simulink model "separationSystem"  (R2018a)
settings: Solver=ode15s  StartTime=0.0  StopTime=180000  RelTol=1e-5
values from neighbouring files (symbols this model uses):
  d_time = 3600*[2,4,18]    [runSimulation.m]    (also in runSimulation_BulkSep.m = 1e6*[1,1,1])
  e_in_val = 0.15    [init_param.m]    (also in init_param_new.m)
  F_in_val = [0.456,0.59]'    [init_param.m]    (also in init_param_new.m)
  ns_tot = ns_o + ns_w + 3    (= 543)    [init_param.m]    (also in runSimulation.m = ns_w + ns_o + 3; RTO.m = 1010; SS.m = 1010)
  rto_sol_time = 6500000    [runSimulation.m]
  t_filter = 2000    [runSimulation.m]
  Y1_case2 = [x_solution(453); x_solution(451); x_solution(452)]    [runSimulation.m]
  Y1_case2_step = 0*(Y1_case2 - Y1.sp)    [runSimulation.m]
  Y1_case3 = [x_solution(453); x_solution(451); x_solution(452)]    [runSimulation.m]
  Y1_case3_step = 0*(Y1_case3 - Y1_case2)    [runSimulation.m]
undefined symbols (not defined in the file or in its folder): c1, cfu, CFU_model_sim, gs1, GS1_model_sim, hc, HC_model_sim, stepTime, U1_step, Y1
libraries: simulink x4

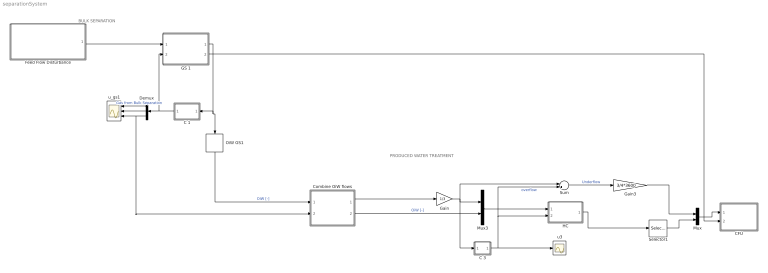
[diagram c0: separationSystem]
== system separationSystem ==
  note: PRODUCED WATER TREATMENT
  note: BULK SEPARATION
  C 1 : Subsystem
  C 3 : Subsystem
  CFU : Subsystem
  Combine OiW flows : Subsystem
  Demux : Demux  Outputs=3
  Feed Flow Disturbance : Subsystem
  GS 1 : Subsystem
  Gain : Gain  Gain=1/3
  Gain3 : Gain  Gain=3/4*3600
  HC : Subsystem
  Mux : Mux  Inputs=2
  Mux3 : Mux  Inputs=2
  OiW GS1 : Selector  InputPortWidth=5  IndexOptions=Index vector (dialog)  Indices=5  OutputSizes=1
  Selector1 : Selector  InputPortWidth=2  IndexOptions=Index vector (dialog)  Indices=[2]  OutputSizes=1
  Sum : Sum  Inputs=|+-
  u3 : Scope
  u_gs1 : Scope  NumInputPorts=3
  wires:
  GS 1/1(Y 1) -> C 1/1(Y 1), OiW GS1/1
  Demux/2 -> u_gs1/2
  C 1/1(U 1) -> GS 1/2(Input), Demux/1
  Demux/1 -> u_gs1/1  "Gas from Bulk Separation"
  C 3/1(U) -> u3/1, Sum/2, HC/2(Input)  "overflow"
  HC/1("Y ") -> Selector1/1
  Mux3/1 -> HC/1(Disturbance)
  Mux/1 -> CFU/1(Disturbance)
  Gain3/1 -> Mux/1
  Sum/1 -> Gain3/1  "Underflow"
  Gain/1 -> Mux3/1, Sum/1, C 3/1(Y)
  OiW GS1/1 -> Combine OiW flows/1("ppm 1 ")  "OiW [-]"
  Demux/3 -> Combine OiW flows/2(flow 1), u_gs1/3
  Feed Flow Disturbance/1(Well Fluids) -> GS 1/1(Disturbance)
  Selector1/1 -> Mux/2
  Combine OiW flows/1(Flow HC feed) -> Gain/1
  Combine OiW flows/2(OiW HC feed) -> Mux3/2  "OiW [-]"
  GS 1/2(Pin) -> CFU/2(Pin)

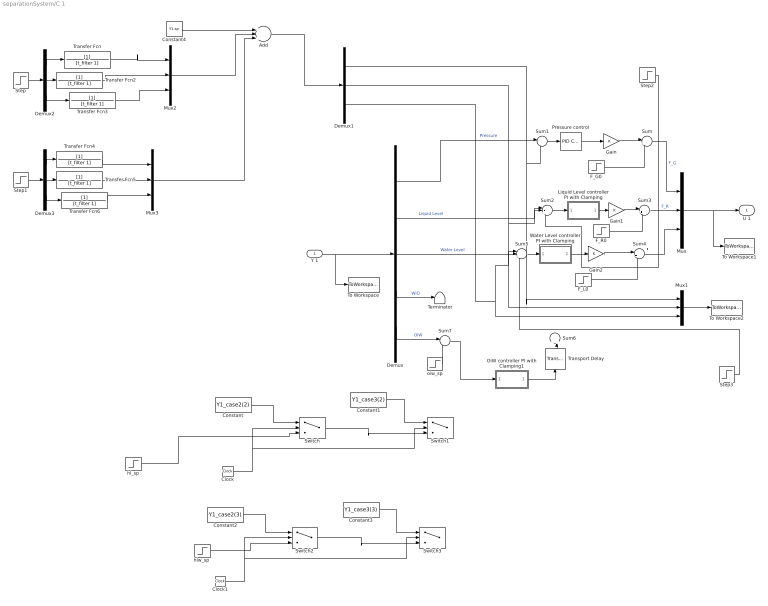
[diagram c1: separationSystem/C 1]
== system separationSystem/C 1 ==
  Y 1 : Inport
  Add : Sum  Inputs=+++
  Clock : Clock
  Clock1 : Clock
  Constant : Constant  Commented=on  Value=Y1_case2(2)
  Constant1 : Constant  Commented=on  Value=Y1_case3(2)
  Constant2 : Constant  Commented=on  Value=Y1_case2(3)
  Constant3 : Constant  Commented=on  Value=Y1_case3(3)
  Constant4 : Constant  Value=Y1.sp
  Demux : Demux  Outputs=5
  Demux1 : Demux  Outputs=3
  Demux2 : Demux  Outputs=3
  Demux3 : Demux  Outputs=3
  F_G0 : Step  Time=stepTime  Before=gs1.U(1)  After=gs1.U(1)*U1_step(1)  SampleTime=0
  F_L0 : Step  Time=stepTime  Before=gs1.U(3)  After=gs1.U(3)*U1_step(3)  SampleTime=0
  F_R0 : Step  Time=stepTime  Before=gs1.U(2)  After=gs1.U(2)*U1_step(2)  SampleTime=0
  Gain : Gain
  Gain1 : Gain
  Gain2 : Gain
  Liquid Level controller PI with Clamping : Subsystem
  Mux{,1..3} (4 alike) : Mux  Inputs=3
  OiW controller PI with Clamping1 : Subsystem  Commented=on
  Pressure control : simulink/Continuous/PID Controller  Controller=PI  TimeDomain=Continuous-time  SampleTime=-1  IntegratorMethod=Forward Euler  FilterMethod=Forward Euler  Form=Parallel  UseFilter=on  ControllerParametersSource=internal  P=-0.1935  I=-0.1935/20  D=0  N=100  InitialConditionSource=internal  InitialConditionForIntegrator=0  InitialConditionForFilter=0  ExternalReset=none  LimitOutput=on  UpperSaturationLimit=inf  LowerSaturationLimit=-gs1.U(1)  LinearizeAsGain=on  AntiWindupMode=none  Kb=1  TrackingMode=off  Kt=1  PParamMin=[]  PParamMax=[]  IParamMin=[]  IParamMax=[]  DParamMin=[]  DParamMax=[]  NParamMin=[]  NParamMax=[]  KbParamMin=[]  KbParamMax=[]  KtParamMin=[]  KtParamMax=[]  POutMin=[]  POutMax=[]  IOutMin=[]  IOutMax=[]  DOutMin=[]  DOutMax=[]  NOutMin=[]  NOutMax=[]  KbOutMin=[]  KbOutMax=[]  KtOutMin=[]  KtOutMax=[]  IntegratorOutMin=[]  IntegratorOutMax=[]  FilterOutMin=[]  FilterOutMax=[]  SumOutMin=[]  SumOutMax=[]  SumI1OutMin=[]  SumI1OutMax=[]  SumI2OutMin=[]  SumI2OutMax=[]  SumI3OutMin=[]  SumI3OutMax=[]  SumDOutMin=[]  SumDOutMax=[]  SaturationOutMin=[]  SaturationOutMax=[]  IntegratorContinuousStateAttributes=''  IntegratorStateMustResolveToSignalObject=off  IntegratorRTWStateStorageClass=Auto  FilterContinuousStateAttributes=''  FilterStateMustResolveToSignalObject=off  FilterRTWStateStorageClass=Auto  DifferentiatorICPrevScaledInput=0  DifferentiatorOutMin=[]  DifferentiatorOutMax=[]  InitialConditionSetting=State (most efficient)  FilterDiffOutCoefMin=[]  FilterDiffOutCoefMax=[]  SumDenOutMin=[]  SumDenOutMax=[]  SumNumOutMin=[]  SumNumOutMax=[]  ReciprocalOutMin=[]  ReciprocalOutMax=[]  DivideOutMin=[]  DivideOutMax=[]  TunerSelectOption=Transfer Function Based (PID Tuner App)
  Step : Step  Time=d_time(2)  After=Y1_case2_step  SampleTime=0
  Step1 : Step  Time=d_time(3)  After=Y1_case3_step  SampleTime=0
  Step2 : Step  Time=126000  After=0.1  SampleTime=0
  Step3 : Step  Time=126000+20000  After=-0.05  SampleTime=0
  Sum : Sum  Inputs=|++
  Sum1 : Sum  Inputs=|-+
  Sum2 : Sum  Inputs=|-++
  Sum3 : Sum  Inputs=|++
  Sum4 : Sum  Inputs=|++
  Sum5 : Sum  Inputs=|-++
  Sum6 : Sum  Commented=on  Inputs=++|
  Sum7 : Sum  Commented=on  Inputs=|-+
  Switch : Switch  Commented=on  Criteria=u2 > Threshold  Threshold=d_time(2)+rto_sol_time
  Switch1 : Switch  Commented=on  Criteria=u2 > Threshold  Threshold=d_time(3)+rto_sol_time
  Switch2 : Switch  Commented=on  Criteria=u2 > Threshold  Threshold=d_time(2)+rto_sol_time
  Switch3 : Switch  Commented=on  Criteria=u2 > Threshold  Threshold=d_time(3)+rto_sol_time
  Terminator : Terminator
  To Workspace : ToWorkspace  VariableName=gs1_Y  SaveFormat=Structure With Time  SampleTime=-1
  To Workspace1 : ToWorkspace  VariableName=gs1_U  SaveFormat=Structure With Time  SampleTime=-1
  To Workspace2 : ToWorkspace  VariableName=gs1_Ysp  SaveFormat=Structure With Time  SampleTime=-1
  Transfer Fcn{,2..6} (6 alike) : TransferFcn  Denominator=[t_filter 1]
  Transport Delay : TransportDelay  Commented=on  DelayTime=0.1
  Water Level controller PI with Clamping : Subsystem
  hl_sp : Step  Commented=on  Time=stepTime  Before=Y1.sp(2)  After=Y1.sp(2)*Y1.step(2)  SampleTime=0
  "hlw_sp " : Step  Commented=on  Time=stepTime  Before=Y1.sp(3)  After=Y1.sp(3)*Y1.step(3)  SampleTime=0
  oiw_sp : Step  Commented=on  Time=stepTime  Before=Y1.sp(4)  After=Y1.sp(4)*Y1.step(4)  SampleTime=0.1
  U 1 : Outport
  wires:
  Sum2/1 -> Liquid Level controller PI with Clamping/1(e)
  Demux1/2 -> Mux1/2, Sum2/2
  Liquid Level controller PI with Clamping/1(delta_u) -> Gain1/1
  Sum5/1 -> Water Level controller PI with Clamping/1(e)
  F_L0/1 -> Sum4/2
  Y 1/1 -> To Workspace/1, Demux/1
  Sum1/1 -> Pressure control/1
  Demux/1 -> Sum1/1  "Pressure"
  Demux1/1 -> Sum1/2, Mux1/1
  Pressure control/1 -> Gain/1
  Mux/1 -> To Workspace1/1, U 1/1
  Demux/2 -> Sum2/1  "Liquid Level"
  Demux/3 -> Sum5/1  "Water Level"
  Water Level controller PI with Clamping/1(delta_u) -> Gain2/1
  Demux/4 -> Terminator/1  "WiO"
  Demux/5 -> Sum7/1  "OiW"
  Sum4/1 -> Mux/3  "F_L"
  Sum3/1 -> Mux/2  "F_R"
  F_R0/1 -> Sum3/2
  F_G0/1 -> Sum/2
  Sum/1 -> Mux/1  "F_G"
  OiW controller PI with Clamping1/1(delta_u) -> Transport Delay/1
  Sum7/1 -> OiW controller PI with Clamping1/1(e)
  oiw_sp/1 -> Sum7/2
  Demux1/3 -> Mux1/3, Sum5/2
  Transport Delay/1 -> Sum6/2
  Mux1/1 -> To Workspace2/1
  Gain/1 -> Sum/1
  Gain1/1 -> Sum3/1
  Gain2/1 -> Sum4/1
  Clock/1 -> Switch/2, Switch1/2
  hl_sp/1 -> Switch/3
  Switch/1 -> Switch1/3
  Constant/1 -> Switch/1
  Constant1/1 -> Switch1/1
  Constant2/1 -> Switch2/1
  Switch2/1 -> Switch3/3
  Constant3/1 -> Switch3/1
  "hlw_sp "/1 -> Switch2/3
  Clock1/1 -> Switch2/2, Switch3/2
  Constant4/1 -> Add/1
  Step/1 -> Demux2/1
  Step1/1 -> Demux3/1
  Mux2/1 -> Add/2
  Mux3/1 -> Add/3
  Add/1 -> Demux1/1
  Demux2/1 -> Transfer Fcn/1
  Demux2/2 -> Transfer Fcn2/1
  Demux2/3 -> Transfer Fcn3/1
  Demux3/1 -> Transfer Fcn4/1
  Demux3/2 -> Transfer Fcn5/1
  Demux3/3 -> Transfer Fcn6/1
  Transfer Fcn/1 -> Mux2/1
  Transfer Fcn2/1 -> Mux2/2
  Transfer Fcn3/1 -> Mux2/3
  Transfer Fcn4/1 -> Mux3/1
  Transfer Fcn5/1 -> Mux3/2
  Transfer Fcn6/1 -> Mux3/3
  Step2/1 -> Sum2/3
  Step3/1 -> Sum5/3

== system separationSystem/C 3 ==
  Y : Inport
  Constant4 : Constant  Value=hc.sp
  Multiply : Product
  To Workspace2 : ToWorkspace  VariableName=hc_U  SaveFormat=Structure With Time  SampleTime=-1
  U : Outport
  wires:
  Y/1 -> Multiply/2  "inflow"
  Multiply/1 -> To Workspace2/1, U/1  "Oil outlet flow (Control input)"
  Constant4/1 -> Multiply/1

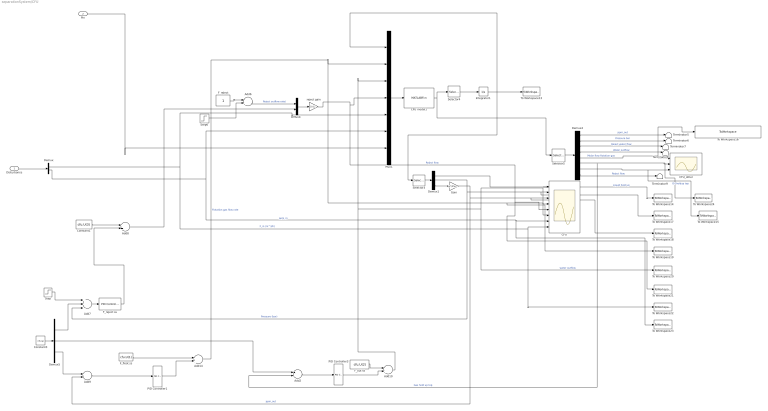
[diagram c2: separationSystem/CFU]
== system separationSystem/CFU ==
  Disturbance : Inport
  Pin : Inport  Port=2
  Add{6,8,10,14} (4 alike) : Sum
  Add2 : Sum  Inputs=+-
  Add7 : Sum  Inputs=++-
  Add9 : Sum  Inputs=+-
  CFU : Scope  NumInputPorts=8
  CFU model1 : MATLABFcn  MATLABFcn=CFU_model_sim(u(1:35),u(36:38),u(39:40),u(41))
  CFU_other : Scope  NumInputPorts=3
  Constant1 : Constant  Value=cfu.U(3)
  Constant3 : Constant  Value=cfu.sp
  Demux : Demux  Outputs=2
  Demux1 : Demux  Outputs=3
  Demux4 : Demux  Outputs=8
  Demux5 : Demux  Outputs=3
  F_float ss : Constant  Value=cfu.U(1)
  F_out ss : Constant  Value=cfu.U(2)
  F_reject : Constant
  F_reject ss : simulink/Continuous/PID Controller  Controller=PI  TimeDomain=Continuous-time  SampleTime=-1  IntegratorMethod=Forward Euler  FilterMethod=Forward Euler  Form=Ideal  UseFilter=on  ControllerParametersSource=internal  P=-36.93/4  I=1/100/4  D=0  N=100  InitialConditionSource=internal  InitialConditionForIntegrator=0  InitialConditionForFilter=0  ExternalReset=none  LimitOutput=off  UpperSaturationLimit=inf  LowerSaturationLimit=0  LinearizeAsGain=on  AntiWindupMode=clamping  Kb=1  TrackingMode=off  Kt=1  PParamMin=[]  PParamMax=[]  IParamMin=[]  IParamMax=[]  DParamMin=[]  DParamMax=[]  NParamMin=[]  NParamMax=[]  KbParamMin=[]  KbParamMax=[]  KtParamMin=[]  KtParamMax=[]  POutMin=[]  POutMax=[]  IOutMin=[]  IOutMax=[]  DOutMin=[]  DOutMax=[]  NOutMin=[]  NOutMax=[]  KbOutMin=[]  KbOutMax=[]  KtOutMin=[]  KtOutMax=[]  IntegratorOutMin=[]  IntegratorOutMax=[]  FilterOutMin=[]  FilterOutMax=[]  SumOutMin=[]  SumOutMax=[]  SumI1OutMin=[]  SumI1OutMax=[]  SumI2OutMin=[]  SumI2OutMax=[]  SumI3OutMin=[]  SumI3OutMax=[]  SumDOutMin=[]  SumDOutMax=[]  SaturationOutMin=[]  SaturationOutMax=[]  IntegratorContinuousStateAttributes=''  IntegratorStateMustResolveToSignalObject=off  IntegratorRTWStateStorageClass=Auto  FilterContinuousStateAttributes=''  FilterStateMustResolveToSignalObject=off  FilterRTWStateStorageClass=Auto  DifferentiatorICPrevScaledInput=0  DifferentiatorOutMin=[]  DifferentiatorOutMax=[]  InitialConditionSetting=State (most efficient)  FilterDiffOutCoefMin=[]  FilterDiffOutCoefMax=[]  SumDenOutMin=[]  SumDenOutMax=[]  SumNumOutMin=[]  SumNumOutMax=[]  ReciprocalOutMin=[]  ReciprocalOutMax=[]  DivideOutMin=[]  DivideOutMax=[]  TunerSelectOption=Transfer Function Based (PID Tuner App)
  Gain : Gain  Gain=pi*(25e-6)^3/6 * 1e10*1e6
  Integrator1 : Integrator  InitialCondition=cfu.x0
  Mux1 : Mux  Inputs=7
  Mux4 : Mux  Inputs=2
  PID Controller1 : simulink/Continuous/PID Controller  Controller=PI  TimeDomain=Continuous-time  SampleTime=-1  IntegratorMethod=Forward Euler  FilterMethod=Forward Euler  Form=Ideal  UseFilter=on  ControllerParametersSource=internal  P=-1.3308/4/5  I=1/100/4/5  D=0  N=100  InitialConditionSource=internal  InitialConditionForIntegrator=0  InitialConditionForFilter=0  ExternalReset=none  LimitOutput=off  UpperSaturationLimit=inf  LowerSaturationLimit=-inf  LinearizeAsGain=on  AntiWindupMode=none  Kb=1  TrackingMode=off  Kt=1  PParamMin=[]  PParamMax=[]  IParamMin=[]  IParamMax=[]  DParamMin=[]  DParamMax=[]  NParamMin=[]  NParamMax=[]  KbParamMin=[]  KbParamMax=[]  KtParamMin=[]  KtParamMax=[]  POutMin=[]  POutMax=[]  IOutMin=[]  IOutMax=[]  DOutMin=[]  DOutMax=[]  NOutMin=[]  NOutMax=[]  KbOutMin=[]  KbOutMax=[]  KtOutMin=[]  KtOutMax=[]  IntegratorOutMin=[]  IntegratorOutMax=[]  FilterOutMin=[]  FilterOutMax=[]  SumOutMin=[]  SumOutMax=[]  SumI1OutMin=[]  SumI1OutMax=[]  SumI2OutMin=[]  SumI2OutMax=[]  SumI3OutMin=[]  SumI3OutMax=[]  SumDOutMin=[]  SumDOutMax=[]  SaturationOutMin=[]  SaturationOutMax=[]  IntegratorContinuousStateAttributes=''  IntegratorStateMustResolveToSignalObject=off  IntegratorRTWStateStorageClass=Auto  FilterContinuousStateAttributes=''  FilterStateMustResolveToSignalObject=off  FilterRTWStateStorageClass=Auto  DifferentiatorICPrevScaledInput=0  DifferentiatorOutMin=[]  DifferentiatorOutMax=[]  InitialConditionSetting=State (most efficient)  FilterDiffOutCoefMin=[]  FilterDiffOutCoefMax=[]  SumDenOutMin=[]  SumDenOutMax=[]  SumNumOutMin=[]  SumNumOutMax=[]  ReciprocalOutMin=[]  ReciprocalOutMax=[]  DivideOutMin=[]  DivideOutMax=[]  TunerSelectOption=Transfer Function Based (PID Tuner App)
  PID Controller3 : simulink/Continuous/PID Controller  Controller=PI  TimeDomain=Continuous-time  SampleTime=-1  IntegratorMethod=Forward Euler  FilterMethod=Forward Euler  Form=Ideal  UseFilter=on  ControllerParametersSource=internal  P=-15.3846  I=1/100  D=0  N=100  InitialConditionSource=internal  InitialConditionForIntegrator=0  InitialConditionForFilter=0  ExternalReset=none  LimitOutput=off  UpperSaturationLimit=inf  LowerSaturationLimit=-inf  LinearizeAsGain=on  AntiWindupMode=none  Kb=1  TrackingMode=off  Kt=1  PParamMin=[]  PParamMax=[]  IParamMin=[]  IParamMax=[]  DParamMin=[]  DParamMax=[]  NParamMin=[]  NParamMax=[]  KbParamMin=[]  KbParamMax=[]  KtParamMin=[]  KtParamMax=[]  POutMin=[]  POutMax=[]  IOutMin=[]  IOutMax=[]  DOutMin=[]  DOutMax=[]  NOutMin=[]  NOutMax=[]  KbOutMin=[]  KbOutMax=[]  KtOutMin=[]  KtOutMax=[]  IntegratorOutMin=[]  IntegratorOutMax=[]  FilterOutMin=[]  FilterOutMax=[]  SumOutMin=[]  SumOutMax=[]  SumI1OutMin=[]  SumI1OutMax=[]  SumI2OutMin=[]  SumI2OutMax=[]  SumI3OutMin=[]  SumI3OutMax=[]  SumDOutMin=[]  SumDOutMax=[]  SaturationOutMin=[]  SaturationOutMax=[]  IntegratorContinuousStateAttributes=''  IntegratorStateMustResolveToSignalObject=off  IntegratorRTWStateStorageClass=Auto  FilterContinuousStateAttributes=''  FilterStateMustResolveToSignalObject=off  FilterRTWStateStorageClass=Auto  DifferentiatorICPrevScaledInput=0  DifferentiatorOutMin=[]  DifferentiatorOutMax=[]  InitialConditionSetting=State (most efficient)  FilterDiffOutCoefMin=[]  FilterDiffOutCoefMax=[]  SumDenOutMin=[]  SumDenOutMax=[]  SumNumOutMin=[]  SumNumOutMax=[]  ReciprocalOutMin=[]  ReciprocalOutMax=[]  DivideOutMin=[]  DivideOutMax=[]  TunerSelectOption=Transfer Function Based (PID Tuner App)
  Selector3 : Selector  InputPortWidth=35  IndexOptions=Index vector (dialog)  Indices=[31 32 33]  OutputSizes=1
  Selector4 : Selector  InputPortWidth=43  IndexOptions=Index vector (dialog)  Indices=[1:35]  OutputSizes=1
  Selector5 : Selector  InputPortWidth=43  IndexOptions=Index vector (dialog)  Indices=[36:43]  OutputSizes=1
  Step : Step  Time=169200+100000  After=-0.05  SampleTime=0
  Step6 : Step  After=0  SampleTime=0
  Terminator{5..9} (5 alike) : Terminator
  To Workspace13 : ToWorkspace  VariableName=x_simulink1  SampleTime=-1
  To Workspace14 : ToWorkspace  VariableName=liq_hold_up1  SampleTime=-1
  To Workspace15 : ToWorkspace  VariableName=oil_hold_up1  SampleTime=-1
  To Workspace16 : ToWorkspace  VariableName=mass_flow_flotation1  SampleTime=-1
  To Workspace17 : ToWorkspace  VariableName=Pressure1  SampleTime=-1
  To Workspace18 : ToWorkspace  VariableName=ppm_out1  SampleTime=-1
  To Workspace19 : ToWorkspace  VariableName=F_flotation1  SampleTime=-1
  To Workspace20 : ToWorkspace  VariableName=F_out1  SampleTime=-1
  To Workspace21 : ToWorkspace  VariableName=F_reject1  SampleTime=-1
  To Workspace22 : ToWorkspace  VariableName=F_in1  SampleTime=-1
  To Workspace23 : ToWorkspace  VariableName=ppm_in1  SampleTime=-1
  To Workspace24 : ToWorkspace  VariableName=gas_hold_up1  SampleTime=-1
  reject gain : Gain  Gain=[0 1]  Multiplication=Matrix(K*u)
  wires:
  Disturbance/1 -> Demux/1
  Add14/1 -> Mux1/2, CFU/6, To Workspace19/1  "Flotation gas flow rate"
  CFU model1/1 -> Selector4/1, Selector5/1
  Demux4/1 -> Terminator5/1  "ppm_out"
  Demux/1 -> Mux1/5, CFU/8, To Workspace22/1  "F_in (m^3/h)"
  Demux4/3 -> Terminator7/1  "Reject water flow"
  Demux1/3 -> Gain/1
  Demux4/4 -> Terminator8/1  "Water outflow"
  Add6/1 -> Mux4/1  "Reject outflow rate)"
  PID Controller1/1 -> Add14/2
  Demux1/1 -> To Workspace14/1, CFU/1  "Liquid hold up"
  F_out ss/1 -> Add10/1
  F_reject/1 -> Add6/1
  Demux4/5 -> To Workspace16/1, CFU_other/1  "Molar flow flotation gas"
  Demux4/7 -> To Workspace15/1, CFU_other/3  "Oil holdup top"
  Demux4/2 -> Terminator6/1  "Pressure bar"
  Selector5/1 -> Demux4/1
  Mux4/1 -> reject gain/1
  Demux1/2 -> Add7/3, CFU/2, To Workspace17/1  "Pressure (bar)"
  reject gain/1 -> CFU/5, To Workspace21/1, Mux1/4  "Reject flow"
  Add8/1 -> Mux4/2
  Step6/1 -> Add6/2
  Gain/1 -> CFU/3, To Workspace18/1, Add9/2  "ppm_out"
  Mux1/1 -> CFU model1/1
  Demux4/8 -> Terminator9/1  "Reject flow"
  Selector3/1 -> Demux1/1
  Integrator1/1 -> To Workspace13/1, Selector3/1, Mux1/1
  F_float ss/1 -> Add14/1
  Selector4/1 -> Integrator1/1
  F_reject ss/1 -> Add8/2
  Demux/2 -> CFU/7, To Workspace23/1, Mux1/6  "ppm_in"
  Constant1/1 -> Add8/1
  Demux4/6 -> Add2/2, To Workspace24/1, CFU_other/2  "Gas hold up top"
  Add9/1 -> PID Controller1/1
  Demux5/1 -> Add7/2
  Demux5/3 -> Add9/1
  Demux5/2 -> Add2/1
  Add7/1 -> F_reject ss/1
  Add10/1 -> Mux1/3, CFU/4, To Workspace20/1  "water outflow"
  Constant3/1 -> Demux5/1
  Add2/1 -> PID Controller3/1
  PID Controller3/1 -> Add10/2
  Pin/1 -> Mux1/7
  Step/1 -> Add7/1

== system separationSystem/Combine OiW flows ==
  "ppm 1 " : Inport
  flow 1 : Inport  Port=2
  Divide : Product  Inputs=*/
  Gain : Gain  Gain=1e-6
  Mux : Mux  Inputs=2
  Product1 : Product
  To Workspace : ToWorkspace  VariableName=D_hc  SaveFormat=Structure With Time  SampleTime=-1
  Flow HC feed : Outport
  OiW HC feed : Outport  Port=2
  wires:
  Product1/1 -> Divide/1  "v1"
  flow 1/1 -> Flow HC feed/1, Mux/1, Divide/2, Product1/2  "v tot"
  "ppm 1 "/1 -> Product1/1
  Divide/1 -> Gain/1
  Mux/1 -> To Workspace/1
  Gain/1 -> Mux/2, OiW HC feed/1

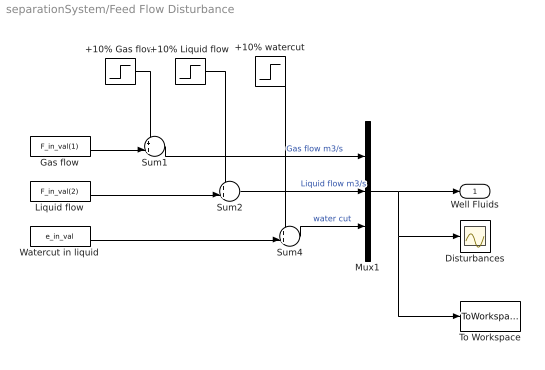
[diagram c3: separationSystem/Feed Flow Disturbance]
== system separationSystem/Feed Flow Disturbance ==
  +10% Gas flow : Step  Time=d_time(1)  After=0.1*F_in_val(1)  SampleTime=0
  +10% Liquid flow : Step  Time=d_time(2)  After=0.1*F_in_val(2)  SampleTime=0
  +10% watercut : Step  Time=d_time(3)  After=0.1*e_in_val  SampleTime=0
  Disturbances : Scope
  Gas flow : Constant  Value=F_in_val(1)
  Liquid flow : Constant  Value=F_in_val(2)
  Mux1 : Mux  Inputs=3
  Sum1 : Sum  Inputs=++|
  Sum2 : Sum  Inputs=++|
  Sum4 : Sum  Inputs=++|
  To Workspace : ToWorkspace  VariableName=simD  SaveFormat=Structure With Time  SampleTime=-1
  Watercut in liquid : Constant  Value=e_in_val
  Well Fluids : Outport
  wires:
  Mux1/1 -> To Workspace/1, Disturbances/1, Well Fluids/1
  Sum2/1 -> Mux1/2  "Liquid flow m3/s"
  Sum4/1 -> Mux1/3  "water cut"
  Liquid flow/1 -> Sum2/2
  Watercut in liquid/1 -> Sum4/2
  +10% Liquid flow/1 -> Sum2/1
  +10% watercut/1 -> Sum4/1
  Sum1/1 -> Mux1/1  "Gas flow m3/s"
  Gas flow/1 -> Sum1/2
  +10% Gas flow/1 -> Sum1/1

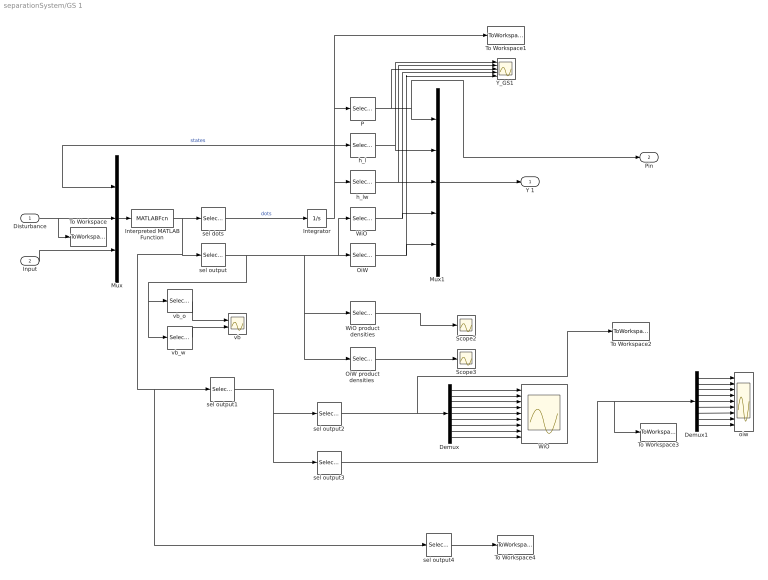
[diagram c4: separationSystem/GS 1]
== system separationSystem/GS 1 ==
  Disturbance : Inport
  Input : Inport  Port=2
  Demux : Demux  Commented=on  Outputs=9
  Demux1 : Demux  Commented=on  Outputs=9
  Integrator : Integrator  InitialCondition=gs1.x0
  Interpreted MATLAB Function : MATLABFcn  MATLABFcn=GS1_model_sim(u(1:ns_tot),u(ns_tot+1:ns_tot+3),u(ns_tot+4:ns_tot+6))
  Mux : Mux  Inputs=3
  Mux1 : Mux  Inputs=5
  OiW : Selector  InputPortWidth=24  IndexOptions=Index vector (dialog)  Indices=[2]  OutputSizes=1
  "OiW product densities " : Selector  InputPortWidth=24  IndexOptions=Index vector (dialog)  Indices=[13:22]  OutputSizes=1
  P : Selector  InputPortWidth=ns_tot  IndexOptions=Index vector (dialog)  Indices=ns_tot  OutputSizes=1
  Scope2 : Scope
  Scope3 : Scope
  To Workspace : ToWorkspace  VariableName=gs1_D  SaveFormat=Structure With Time  SampleTime=-1
  To Workspace1 : ToWorkspace  VariableName=xSol_gs1  SaveFormat=Structure With Time  SampleTime=-1
  To Workspace2 : ToWorkspace  VariableName=wio  SampleTime=-1
  To Workspace3 : ToWorkspace  VariableName=oiw  SampleTime=-1
  To Workspace4 : ToWorkspace  VariableName=rho_all  SampleTime=-1
  WiO : Scope  NumInputPorts=9
  "WiO " : Selector  InputPortWidth=24  IndexOptions=Index vector (dialog)  Indices=[1]  OutputSizes=1
  WiO product densities : Selector  InputPortWidth=24  IndexOptions=Index vector (dialog)  Indices=[3:12]  OutputSizes=1
  "Y_GS1 " : Scope  NumInputPorts=5
  h_l : Selector  InputPortWidth=ns_tot  IndexOptions=Index vector (dialog)  Indices=[ns_tot-2]  OutputSizes=1
  h_lw : Selector  InputPortWidth=ns_tot  IndexOptions=Index vector (dialog)  Indices=[ns_tot-1]  OutputSizes=1
  oiw : Scope  NumInputPorts=9
  sel dots : Selector  InputPortWidth=ns_tot+24+18+180+66+300  IndexOptions=Index vector (dialog)  Indices=[1:ns_tot]  OutputSizes=1
  sel output : Selector  InputPortWidth=ns_tot+24+18+180+66+300  IndexOptions=Index vector (dialog)  Indices=[ns_tot+1:ns_tot+24]  OutputSizes=1
  sel output1 : Selector  InputPortWidth=ns_tot+24+18+180+66+300  IndexOptions=Index vector (dialog)  Indices=[ns_tot+24+1:ns_tot+24+18+6]  OutputSizes=1
  sel output2 : Selector  InputPortWidth=24  IndexOptions=Index vector (dialog)  Indices=[1:12]  OutputSizes=1
  sel output3 : Selector  InputPortWidth=24  IndexOptions=Index vector (dialog)  Indices=[13:24]  OutputSizes=1
  sel output4 : Selector  InputPortWidth=ns_tot+24+18+180+66+300  IndexOptions=Index vector (dialog)  Indices=[ns_tot+24+18+6+1:ns_tot+24+18+180+66+300]  OutputSizes=1
  vb : Scope  NumInputPorts=2
  vb_o : Selector  InputPortWidth=24  IndexOptions=Index vector (dialog)  Indices=[23]  OutputSizes=1
  "vb_w " : Selector  InputPortWidth=24  IndexOptions=Index vector (dialog)  Indices=[24]  OutputSizes=1
  Y 1 : Outport
  Pin : Outport  Port=2
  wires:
  Mux/1 -> Interpreted MATLAB Function/1
  Integrator/1 -> To Workspace1/1, P/1, Mux/1, h_l/1, h_lw/1  "states"
  Interpreted MATLAB Function/1 -> sel output4/1, sel output1/1, sel output/1, sel dots/1
  sel output/1 -> vb_o/1, "vb_w "/1, "OiW product densities "/1, WiO product densities/1, "WiO "/1, OiW/1
  "vb_w "/1 -> vb/2
  vb_o/1 -> vb/1
  Input/1 -> Mux/3
  Disturbance/1 -> To Workspace/1, Mux/2
  Mux1/1 -> Y 1/1
  OiW/1 -> Mux1/5, "Y_GS1 "/5
  WiO product densities/1 -> Scope2/1
  P/1 -> "Y_GS1 "/3, Pin/1, Mux1/1
  h_lw/1 -> "Y_GS1 "/2, Mux1/3
  "WiO "/1 -> Mux1/4, "Y_GS1 "/4
  "OiW product densities "/1 -> Scope3/1
  sel dots/1 -> Integrator/1  "dots"
  h_l/1 -> "Y_GS1 "/1, Mux1/2
  sel output1/1 -> sel output3/1, sel output2/1
  sel output2/1 -> To Workspace2/1, Demux/1
  Demux/1 -> WiO/1
  Demux/2 -> WiO/2
  Demux/3 -> WiO/3
  Demux/4 -> WiO/4
  Demux/5 -> WiO/5
  Demux/6 -> WiO/6
  Demux/7 -> WiO/7
  Demux/8 -> WiO/8
  Demux/9 -> WiO/9
  Demux1/7 -> oiw/7
  Demux1/1 -> oiw/1
  Demux1/4 -> oiw/4
  Demux1/6 -> oiw/6
  Demux1/9 -> oiw/9
  Demux1/3 -> oiw/3
  sel output3/1 -> To Workspace3/1, Demux1/1
  Demux1/8 -> oiw/8
  Demux1/5 -> oiw/5
  Demux1/2 -> oiw/2
  sel output4/1 -> To Workspace4/1

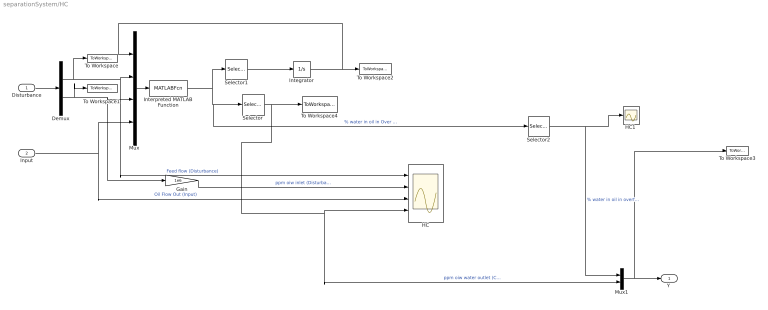
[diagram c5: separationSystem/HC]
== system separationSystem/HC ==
  Disturbance : Inport
  Input : Inport  Port=2
  Demux : Demux  Outputs=2
  Gain : Gain  Gain=1e6
  HC : Scope  NumInputPorts=4
  "HC1 " : Scope
  Integrator : Integrator  InitialCondition=hc.x0
  Interpreted MATLAB Function : MATLABFcn  MATLABFcn=HC_model_sim(u(1:432),u(433),u(434),u(435))
  Mux : Mux
  Mux1 : Mux  Inputs=2
  Selector : Selector  InputPortWidth=436  IndexOptions=Index vector (dialog)  Indices=[435]  OutputSizes=1
  Selector1 : Selector  InputPortWidth=436  IndexOptions=Index vector (dialog)  Indices=[1:432]  OutputSizes=1
  Selector2 : Selector  InputPortWidth=436  IndexOptions=Index vector (dialog)  Indices=[436]  OutputSizes=1
  To Workspace : ToWorkspace  VariableName=F_in_sim  SampleTime=-1
  To Workspace1 : ToWorkspace  VariableName=e_in_sim  SampleTime=-1
  To Workspace2 : ToWorkspace  VariableName=xSol_hc  SaveFormat=Structure With Time  SampleTime=-1
  To Workspace3 : ToWorkspace  VariableName=hc_Y  SaveFormat=Structure With Time  SampleTime=-1
  To Workspace4 : ToWorkspace  VariableName=e_out_sim  SampleTime=-1
  "Y " : Outport
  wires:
  Integrator/1 -> Mux/1, To Workspace2/1
  Selector/1 -> Mux1/2, HC/4, To Workspace4/1  "ppm oiw water outlet (CV)"
  Interpreted MATLAB Function/1 -> Selector1/1, Selector2/1, Selector/1  "% water in oil in Over flow"
  Mux/1 -> Interpreted MATLAB Function/1
  Gain/1 -> HC/2  "ppm oiw inlet (Disturbance)"
  Disturbance/1 -> Demux/1
  Input/1 -> Mux/4, HC/3  "Oil Flow Out (Input)"
  Selector1/1 -> Integrator/1
  Demux/1 -> To Workspace/1, HC/1, Mux/2  "Feed flow (Disturbance)"
  Demux/2 -> To Workspace1/1, Gain/1, Mux/3
  Selector2/1 -> "HC1 "/1, Mux1/1  "% water in oil in overflow"
  Mux1/1 -> To Workspace3/1, "Y "/1

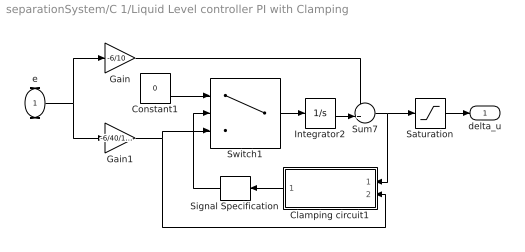
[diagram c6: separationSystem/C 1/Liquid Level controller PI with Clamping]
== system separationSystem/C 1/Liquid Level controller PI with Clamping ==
  e : Inport
  Clamping circuit1 : Subsystem
  Constant1 : Constant  Value=0
  Gain : Gain  Gain=-6/10
  Gain1 : Gain  Gain=-6/40/100
  Integrator2 : Integrator
  Saturation : Saturate  UpperLimit=inf  LowerLimit=-gs1.U(2)
  Signal Specification : SignalSpecification  Dimensions=1
  Sum7 : Sum  Inputs=++|
  Switch1 : Switch  Criteria=u2 > Threshold
  delta_u : Outport
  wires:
  Sum7/1 -> Clamping circuit1/1(preSat), Saturation/1
  Integrator2/1 -> Sum7/2
  Saturation/1 -> delta_u/1
  Switch1/1 -> Integrator2/1
  Constant1/1 -> Switch1/1
  e/1 -> Gain1/1, Gain/1
  Gain1/1 -> Clamping circuit1/2(preIntegrator), Switch1/3
  Gain/1 -> Sum7/1
  Clamping circuit1/1(Clamp) -> Signal Specification/1
  Signal Specification/1 -> Switch1/2

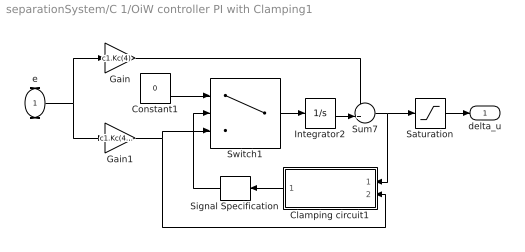
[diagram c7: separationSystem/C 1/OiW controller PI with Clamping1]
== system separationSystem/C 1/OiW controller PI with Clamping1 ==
  e : Inport
  Clamping circuit1 : Subsystem
  Constant1 : Constant  Value=0
  Gain : Gain  Gain=c1.Kc(4)
  Gain1 : Gain  Gain=c1.Kc(4)/c1.taui(4)
  Integrator2 : Integrator
  Saturation : Saturate  UpperLimit=4-Y1.sp(3)  LowerLimit=-Y1.sp(3)
  Signal Specification : SignalSpecification  Dimensions=1
  Sum7 : Sum  Inputs=++|
  Switch1 : Switch  Criteria=u2 > Threshold
  delta_u : Outport
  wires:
  Sum7/1 -> Clamping circuit1/1(preSat), Saturation/1
  Integrator2/1 -> Sum7/2
  Saturation/1 -> delta_u/1
  Switch1/1 -> Integrator2/1
  Constant1/1 -> Switch1/1
  e/1 -> Gain1/1, Gain/1
  Gain1/1 -> Clamping circuit1/2(preIntegrator), Switch1/3
  Gain/1 -> Sum7/1
  Clamping circuit1/1(Clamp) -> Signal Specification/1
  Signal Specification/1 -> Switch1/2

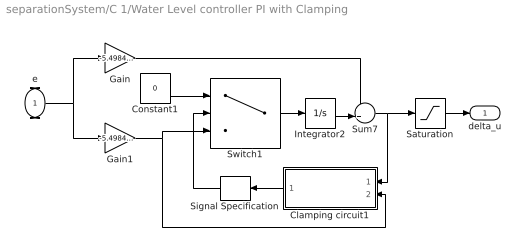
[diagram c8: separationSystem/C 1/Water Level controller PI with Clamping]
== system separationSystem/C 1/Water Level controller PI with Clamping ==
  e : Inport
  Clamping circuit1 : Subsystem
  Constant1 : Constant  Value=0
  Gain : Gain  Gain=-5.4984/200
  Gain1 : Gain  Gain=-5.4984/40/40000
  Integrator2 : Integrator
  Saturation : Saturate  UpperLimit=inf  LowerLimit=-gs1.U(3)
  Signal Specification : SignalSpecification  Dimensions=1
  Sum7 : Sum  Inputs=++|
  Switch1 : Switch  Criteria=u2 > Threshold
  delta_u : Outport
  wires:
  Sum7/1 -> Clamping circuit1/1(preSat), Saturation/1
  Integrator2/1 -> Sum7/2
  Saturation/1 -> delta_u/1
  Switch1/1 -> Integrator2/1
  Constant1/1 -> Switch1/1
  e/1 -> Gain1/1, Gain/1
  Gain1/1 -> Clamping circuit1/2(preIntegrator), Switch1/3
  Gain/1 -> Sum7/1
  Clamping circuit1/1(Clamp) -> Signal Specification/1
  Signal Specification/1 -> Switch1/2

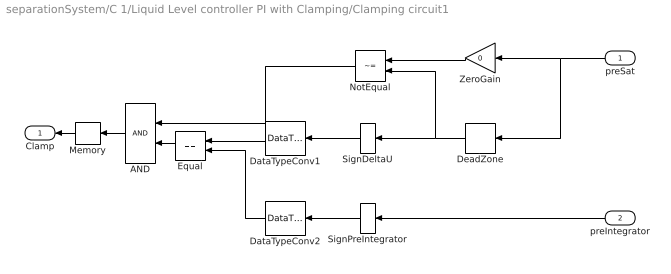
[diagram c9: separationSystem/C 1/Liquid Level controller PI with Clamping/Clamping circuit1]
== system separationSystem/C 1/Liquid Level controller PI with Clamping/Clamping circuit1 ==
  preSat : Inport  DisableCoverage=on
  preIntegrator : Inport  DisableCoverage=on  Port=2
  AND : Logic  DisableCoverage=on
  DataTypeConv1 : DataTypeConversion  DisableCoverage=on  OutDataTypeStr=int8
  DataTypeConv2 : DataTypeConversion  DisableCoverage=on  OutDataTypeStr=int8
  DeadZone : DeadZone  DisableCoverage=on  LowerValue=-gs1.U(2)  UpperValue=inf
  Equal : RelationalOperator  DisableCoverage=on  Operator===
  Memory : Memory  DisableCoverage=on
  NotEqual : RelationalOperator  DisableCoverage=on  Operator=~=
  SignDeltaU : Signum  DisableCoverage=on
  SignPreIntegrator : Signum  DisableCoverage=on
  ZeroGain : Gain  DisableCoverage=on  Gain=0
  Clamp : Outport  DisableCoverage=on
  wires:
  preSat/1 -> ZeroGain/1, DeadZone/1
  preIntegrator/1 -> SignPreIntegrator/1
  ZeroGain/1 -> NotEqual/1
  DeadZone/1 -> NotEqual/2, SignDeltaU/1
  SignDeltaU/1 -> DataTypeConv1/1
  DataTypeConv1/1 -> Equal/1
  SignPreIntegrator/1 -> DataTypeConv2/1
  DataTypeConv2/1 -> Equal/2
  NotEqual/1 -> AND/1
  Equal/1 -> AND/2
  AND/1 -> Memory/1
  Memory/1 -> Clamp/1

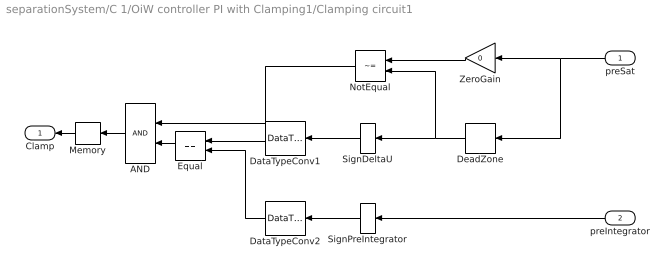
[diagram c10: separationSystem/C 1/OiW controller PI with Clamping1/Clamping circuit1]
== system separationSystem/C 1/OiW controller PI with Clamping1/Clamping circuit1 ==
  preSat : Inport  DisableCoverage=on
  preIntegrator : Inport  DisableCoverage=on  Port=2
  AND : Logic  DisableCoverage=on
  DataTypeConv1 : DataTypeConversion  DisableCoverage=on  OutDataTypeStr=int8
  DataTypeConv2 : DataTypeConversion  DisableCoverage=on  OutDataTypeStr=int8
  DeadZone : DeadZone  DisableCoverage=on  LowerValue=-Y1.sp(3)  UpperValue=4-Y1.sp(3)
  Equal : RelationalOperator  DisableCoverage=on  Operator===
  Memory : Memory  DisableCoverage=on
  NotEqual : RelationalOperator  DisableCoverage=on  Operator=~=
  SignDeltaU : Signum  DisableCoverage=on
  SignPreIntegrator : Signum  DisableCoverage=on
  ZeroGain : Gain  DisableCoverage=on  Gain=0
  Clamp : Outport  DisableCoverage=on
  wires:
  preSat/1 -> ZeroGain/1, DeadZone/1
  preIntegrator/1 -> SignPreIntegrator/1
  ZeroGain/1 -> NotEqual/1
  DeadZone/1 -> NotEqual/2, SignDeltaU/1
  SignDeltaU/1 -> DataTypeConv1/1
  DataTypeConv1/1 -> Equal/1
  SignPreIntegrator/1 -> DataTypeConv2/1
  DataTypeConv2/1 -> Equal/2
  NotEqual/1 -> AND/1
  Equal/1 -> AND/2
  AND/1 -> Memory/1
  Memory/1 -> Clamp/1

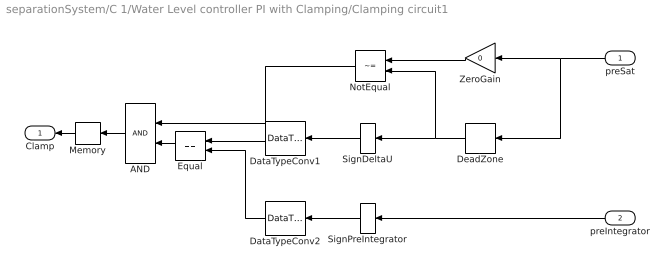
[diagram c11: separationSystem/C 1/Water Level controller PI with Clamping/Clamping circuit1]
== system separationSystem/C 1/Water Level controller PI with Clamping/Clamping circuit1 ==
  preSat : Inport  DisableCoverage=on
  preIntegrator : Inport  DisableCoverage=on  Port=2
  AND : Logic  DisableCoverage=on
  DataTypeConv1 : DataTypeConversion  DisableCoverage=on  OutDataTypeStr=int8
  DataTypeConv2 : DataTypeConversion  DisableCoverage=on  OutDataTypeStr=int8
  DeadZone : DeadZone  DisableCoverage=on  LowerValue=-gs1.U(3)  UpperValue=inf
  Equal : RelationalOperator  DisableCoverage=on  Operator===
  Memory : Memory  DisableCoverage=on
  NotEqual : RelationalOperator  DisableCoverage=on  Operator=~=
  SignDeltaU : Signum  DisableCoverage=on
  SignPreIntegrator : Signum  DisableCoverage=on
  ZeroGain : Gain  DisableCoverage=on  Gain=0
  Clamp : Outport  DisableCoverage=on
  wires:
  preSat/1 -> ZeroGain/1, DeadZone/1
  preIntegrator/1 -> SignPreIntegrator/1
  ZeroGain/1 -> NotEqual/1
  DeadZone/1 -> NotEqual/2, SignDeltaU/1
  SignDeltaU/1 -> DataTypeConv1/1
  DataTypeConv1/1 -> Equal/1
  SignPreIntegrator/1 -> DataTypeConv2/1
  DataTypeConv2/1 -> Equal/2
  NotEqual/1 -> AND/1
  Equal/1 -> AND/2
  AND/1 -> Memory/1
  Memory/1 -> Clamp/1
